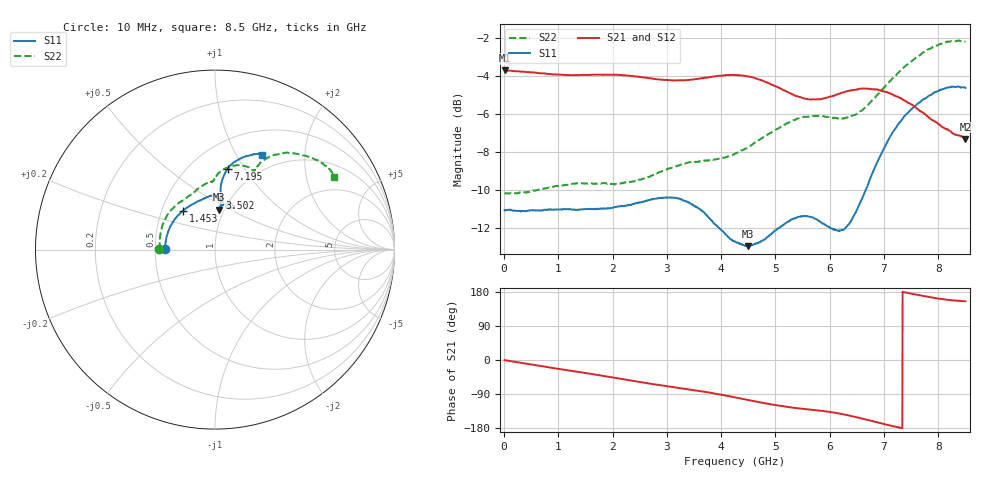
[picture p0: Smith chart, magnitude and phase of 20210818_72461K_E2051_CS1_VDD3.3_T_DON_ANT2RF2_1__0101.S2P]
!Agilent Technologies,E5071C,MY46417908,A.11.23
!Date: Wed Aug 18 14:27:26 2021
!Data & Calibration Information:
!Freq	S11:SOLT2(ON)	S21:SOLT2(ON)	S12:SOLT2(ON)	S22:SOLT2(ON)
!PortZ  Port1:50+j0  Port2:50+j0
!Above PortZ is port z conversion or system Z0 setting when saving the data.
!When reading, reference impedance value at option line is always used.
# Hz S dB R 50
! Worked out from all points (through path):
!   1601 points, 10 MHz to 8.5 GHz, reference 50 ohm
!   highest |S21| = -3.68 dB at 10 MHz (marker M1); lowest = -7.3 dB at 8.5 GHz (marker M2)
!   group delay of S21, straight-line fit = 67.7 ps
!   lowest |S11| = -13.0 dB at 4.499 GHz (marker M3), VSWR 1.58, Z = 47.2 + j22.2 ohm
!   |S11| at or under -10 dB: start of sweep to 6.665 GHz
!   |S22| runs from -10.2 to -2.1 dB; largest |S21 - S12| = 0.0025
!   S11 on the Smith chart (normalised r, x): 10 MHz: 0.56, +0.00; 1.453 GHz: 0.64, +0.30; 3.502 GHz: 0.89, +0.55; 7.195 GHz: 0.74, +0.84; 8.5 GHz: 0.79, +1.28
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1e7  -11.08 179.5  -3.68 -0.4  -3.68 -0.4  -10.16 179.8
7.847125e8  -11.06 155.2  -3.87 -18.6  -3.86 -18.6  -9.91 159.2
1.426769e9  -11.04 130.7  -3.93 -32.7  -3.93 -32.7  -9.65 139.5
1.4533e9  -11.03 129.7  -3.93 -33.3  -3.93 -33.2  -9.66 138.7
2.190869e9  -10.86 106.9  -3.96 -50.7  -3.96 -50.7  -9.65 118.8
2.843538e9  -10.45 94.9  -4.16 -65.7  -4.16 -65.8  -9.09 106.0
3.501512e9  -10.84 84.9  -4.17 -79.5  -4.16 -79.5  -8.54 95.7
3.936625e9  -11.95 81.8  -3.98 -89.8  -3.98 -89.8  -8.37 91.8
4.255e9  -12.74 82.4  -3.94 -98.6  -3.93 -98.6  -8.10 90.2
4.499088e9  -12.98 84.2  -4.02 -105.6  -4.01 -105.6  -7.74 88.9
5.040325e9  -12.04 81.4  -4.57 -119.9  -4.58 -119.9  -6.78 82.3
5.422375e9  -11.43 72.8  -5.08 -127.5  -5.09 -127.6  -6.23 74.5
5.671769e9  -11.45 67.6  -5.23 -131.3  -5.23 -131.4  -6.11 69.7
5.947694e9  -11.91 66.2  -5.13 -135.9  -5.14 -135.9  -6.15 65.6
6.297906e9  -11.98 75.1  -4.80 -144.6  -4.80 -144.8  -6.19 63.2
6.706488e9  -9.71 84.6  -4.66 -158.6  -4.65 -158.7  -5.51 62.7
7.088538e9  -7.31 82.5  -4.88 -172.0  -4.89 -172.1  -4.33 59.1
7.194662e9  -6.83 81.1  -5.03 -175.4  -5.03 -175.5  -4.03 57.2
7.449362e9  -5.91 76.7  -5.42 176.8  -5.42 176.8  -3.35 52.4
7.831412e9  -5.03 69.7  -6.20 166.1  -6.17 166.0  -2.57 43.3
8.197544e9  -4.59 65.2  -6.87 158.4  -6.84 158.5  -2.18 35.6
8.5e9  -4.61 63.8  -7.31 154.9  -7.27 155.0  -2.19 31.4
